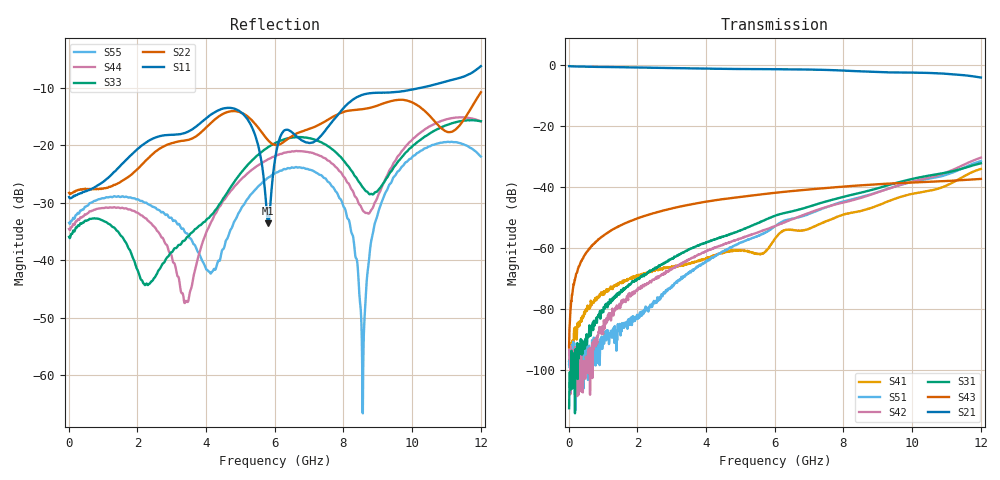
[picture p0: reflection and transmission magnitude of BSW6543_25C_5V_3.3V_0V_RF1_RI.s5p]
! Agilent Technologies	N5230C	MY49001333	A.09.33.09
!	Test time	=	2026-05-28 10:00
!	Product	=	BSW6543
!	Temp	=	25C
!	Logic	=	RF1
!	Port1	=	RFC
!	Port2	=	RF1
!	Port3	=	RF2
!	Port4	=	RF3
!	Port5	=	RF4
!S5P File: Measurements: <S11,S12,S13,S14,S15>,
!<S21,S22,S23,S24,S25>,
!<S31,S32,S33,S34,S35>,
!<S41,S42,S43,S44,S45>,
!<S51,S52,S53,S54,S55>;
# HZ S RI R 50
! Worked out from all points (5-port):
!   1201 points, 10 MHz to 12.01 GHz, reference 50 ohm
!   strongest paths, dB at 10 MHz, 3.01 GHz, 6.01 GHz, 9.01 GHz, 12.01 GHz:
!     S21: -0.5, -1.1, -1.5, -2.4, -4.2
!     S43: -92.5, -47.0, -41.9, -39.1, -37.4
!     S31: -112.4, -63.5, -49.4, -40.4, -32.2
!     S42: -92.0, -66.8, -52.8, -41.7, -30.4
!     S51: -97.9, -72.8, -52.9, -41.7, -31.5
!     S41: -97.1, -66.0, -57.0, -46.0, -34.1
!   lowest |S11| = -33.6 dB at 5.81 GHz (marker M1), VSWR 1.04, Z = 48 + j0.467 ohm
!   |S11| at or under -10 dB: start of sweep to 10.28 GHz
